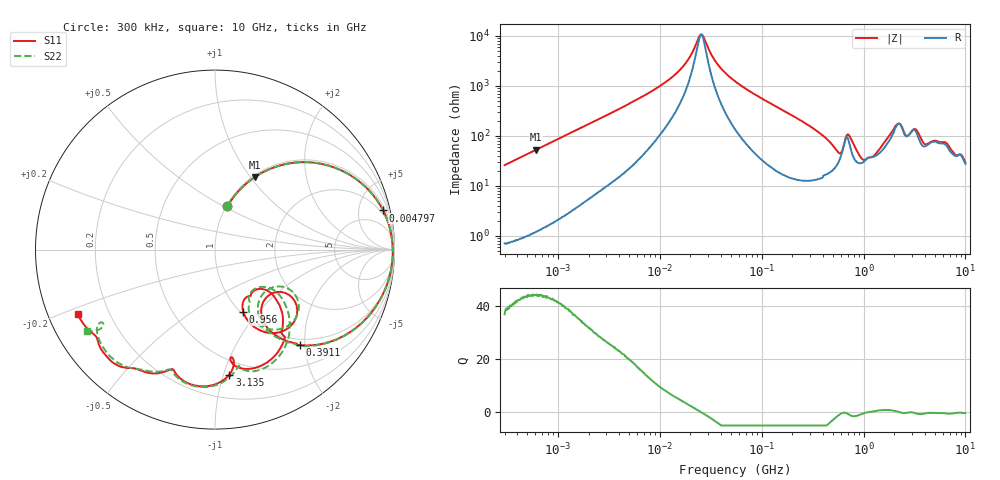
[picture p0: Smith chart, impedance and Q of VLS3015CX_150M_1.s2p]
! S-Parameter Data Generated by TDK Corporation
! Copyright(C) 2020 TDK Corporation.
! All Rights Reserved.
! TDK P/N: VLS3015CX-150M-1 (Inductor)
! Property: L=15uH at 1MHz
! Size(LxWxT): 3x3x1.5mm
! Model Type: s2p (Touchstone File Format Version 1.0)
! Frequency: DC=Yes Start=0.3MHz Stop=10000MHz 802points Log-sweep
! Model Generated on Aug. 18, 2020
! Port Assignments:
!  1 ---@@@--- 2
! Applicable Conditions:
!  Temperature = 25 degC
!  DC Bias Current = 0 A
!  Small Signal Operation
! Terms and conditions regarding TDK Simulation Models
! (1)This simulation model is being provided solely for informational purposes. Please refer to the specifications of the products in terms of detailed characteristics of such products.
! (2)In no event shall TDK Corporation of any of its subsidiaries be liable for any loss or damage arising, directly or indirectly,
!  From any information contained in this simulation model, including, but not limited to loss or damages arising from any inaccuracies, omissions or errors in connection with such information.
! (3)Any and all copyrights on this simulation model are owned by TDK Corporation.
!  Duplication or redistribution of this simulation model without prior written permission from TDK Corporation is prohibited.
! (4)This simulation model is subject to any modification or change without any prior notice.
! (5)Neither TDK Corporation nor any of its subsidiaries shall make any warranty, express or implied,
!  Including but not limited to the correctness, implied warranties of merchantability and fitness for a particular purpose with respect to this simulation models.
! (6)The use of this simulation model shall be deemed to have consented to the terms and conditions hereof.
# Hz S MA R 50
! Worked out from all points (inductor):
!   801 points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, 300 kHz to 10 GHz, reference 50 ohm
!   read as one part in series: L = 13.8 uH near 318.3 kHz
!   highest Q = 44 at 610.3 kHz (marker M1), where L = 13.7 uH
!   self-resonance near 25.36 MHz
!   S11 on the Smith chart (normalised r, x): 300 kHz: 1.01, +0.52; 4.797 MHz: 1.45, +8.45; 391.1 MHz: 0.88, -1.90; 956 MHz: 1.03, -0.84; 3.135 GHz: 0.38, -1.05; 10 GHz: 0.09, -0.22
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300000  0.2501 74.0  0.9615 -14.4  0.9612 -14.4  0.2498 74.0
610333  0.4619 61.2  0.8763 -27.5  0.8764 -27.5  0.4619 61.2
1713600  0.8158 33.6  0.5548 -54.7  0.5547 -54.7  0.8159 33.6
4796912  0.9619 13.1  0.2295 -74.0  0.2294 -74.1  0.962 13.1
9671944  0.9842 5.7  0.1038 -78.6  0.1038 -78.6  0.9842 5.7
1.694973e7  0.9893 1.8  0.0402 -74.0  0.04019 -74.0  0.9893 1.8
2.567637e7  0.9906 -0.7  0.009254 2.3  0.009257 2.3  0.9907 -0.7
3.642588e7  0.9904 -2.9  0.03514 72.5  0.03515 72.5  0.9905 -3.0
5.477226e7  0.988 -6.0  0.07961 77.7  0.0796 77.7  0.988 -6.1
1.563148e8  0.9469 -20.3  0.2767 66.8  0.2766 66.8  0.9469 -20.4
3.126428e8  0.8099 -39.9  0.5234 45.2  0.5233 45.2  0.8093 -40.2
3.910695e8  0.7117 -48.4  0.6188 34.1  0.6187 34.1  0.7101 -48.9
5.414944e8  0.4692 -55.6  0.7197 10.5  0.7195 10.5  0.457 -57.0
6.325141e8  0.4198 -34.2  0.6183 -6.8  0.6182 -6.8  0.3891 -32.2
7.318083e8  0.5986 -46.5  0.5198 8.8  0.5197 8.8  0.5917 -42.8
9.560117e8  0.3809 -65.6  0.7232 -6.8  0.7232 -6.7  0.4034 -61.5
1.339606e9  0.3178 -45.1  0.6846 -32.0  0.6846 -32.1  0.3104 -45.5
1.767019e9  0.4817 -41.2  0.5107 -55.7  0.5106 -55.7  0.4928 -37.8
2.294622e9  0.6956 -67.6  0.2913 -45.4  0.2911 -45.4  0.712 -64.8
3.135132e9  0.7005 -83.4  0.285 -52.9  0.2849 -52.8  0.7474 -88.1
6.576072e9  0.8349 -128.5  0.2173 -76.4  0.2176 -76.3  0.8268 -129.4
1e10  0.8456 -154.7  0.1836 -86.9  0.1836 -86.9  0.846 -147.7
